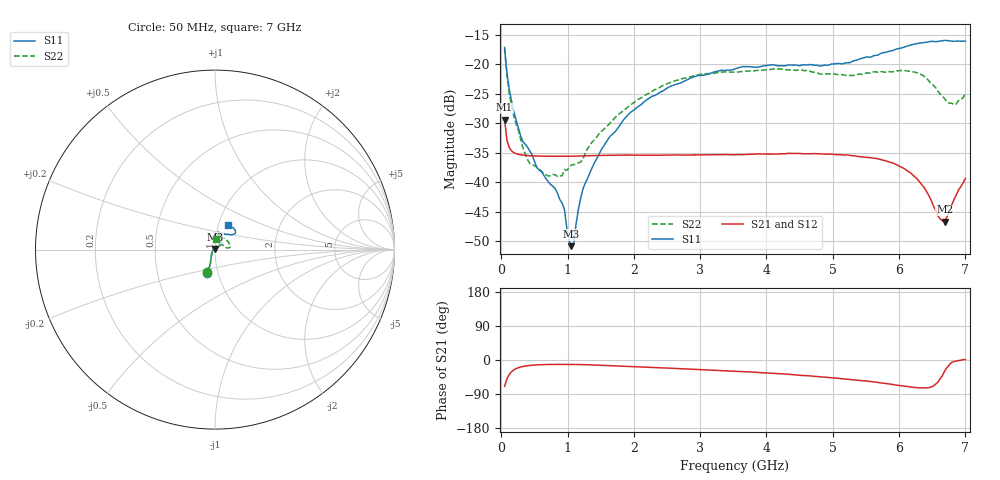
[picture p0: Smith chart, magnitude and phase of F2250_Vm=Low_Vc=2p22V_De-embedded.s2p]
! Integrated Device Technology
! Corporate Headquarters
! 6024 Silver Creek Valley Road
! San Jose, CA 95138  USA
! Phone:  1-408-284-8200
! Toll Free:  1-800-223-1366
! Webpage:  http://www.idt.com/
! Timing and RF Division
! 515 Groton Road, Suite 102
! Westford, MA 01886-6024
! Device:  F2250
! Description: Voltage Variable RF Attenuator
! Frequency:  50.0 -  6000.00 MHz
! Package:  3x3 mm Thin QFN Plastic Package: 16 pin
! Ports:  2 RF, 3 DC
!  Pin  1  = GND
!  Pin  2  = NC
!  Pin  3  = RF1  = Port 1
!  Pin  4  = NC
!  Pin  5  = GND
!  Pin  6  = GND
!  Pin  7  = GND
!  Pin  8  = GND
!  Pin  9  = NC
!  Pin 10  = RF2  = Port 2
!  Pin 11  = NC
!  Pin 12  = GND
!  Pin 13  = GND
!  Pin 14  = VCNTRL
!  Pin 15  = VDD
!  Pin 16  = VMODE
! Vcntrl:  2.220 Volts
! Vmode:  +0.000 Volts
! Vdd:  +3.30  Volts
! Current:  1.177 mA
! Data:  The device was measured on a the F2250 evaluation board which has
!  individual transmission lines to the RF pins.  Data was collected
!  using a calibrated network analyzer.  The evaluation board was
!  de-embedded using a TRL calibration technique.
!  The reference plane is the edge of the package pin.
! Misc:  SN 10
!  Action Tracker AT0258
! Date Measured:  2014-11-26
! Date:  2015-10-15  MJV
! Note:
!  Integrated Device Technology supplies this data as a sample of measured
!  data at the package pin for this product.  Your particular data for this
!  product may vary.
!  Data was taken at 25 degrees C.
!  Integrated Device Technology reserves the right to change this data at anytime.
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# GHz S dB R 50
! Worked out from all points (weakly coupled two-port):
!   201 points, 50 MHz to 7 GHz, reference 50 ohm
!   highest |S21| = -29.39 dB at 50 MHz (marker M1); lowest = -46.7 dB at 6.687 GHz (marker M2)
!   lowest |S11| = -50.8 dB at 1.058 GHz (marker M3), VSWR 1.01, Z = 49.8 + j0.239 ohm
!   |S11| at or under -10 dB: start of sweep to end of sweep
!   |S22| runs from -39.0 to -17.4 dB; largest |S21 - S12| = 5.9e-05
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0.05  -17.18 -108.6  -29.39 -69.5  -29.38 -69.5  -17.38 -110.5
0.08475  -21.44 -107.4  -32.86 -50.1  -32.87 -50.1  -21.91 -109.0
0.15425  -26.23 -116.6  -34.68 -31.0  -34.68 -30.9  -27.12 -120.1
0.29325  -32.19 -127.8  -35.35 -18.4  -35.35 -18.4  -32.74 -133.5
0.3975  -34.09 -141.8  -35.48 -14.9  -35.48 -15.0  -36.19 -157.2
0.71025  -39.94 -168.7  -35.59 -11.8  -35.59 -11.8  -38.94 153.7
0.91875  -43.54 158.0  -35.61 -11.6  -35.60 -11.5  -38.87 127.1
1.023  -49.91 144.0  -35.59 -11.6  -35.59 -11.6  -37.54 108.4
1.05775  -50.81 123.5  -35.59 -11.7  -35.59 -11.7  -37.07 103.0
1.0925  -50.38 89.2  -35.58 -11.8  -35.58 -11.7  -37.00 98.4
1.162  -44.67 56.8  -35.56 -11.9  -35.56 -11.9  -36.69 87.1
1.2315  -41.13 44.4  -35.53 -12.2  -35.53 -12.2  -36.06 77.7
1.6485  -32.11 42.0  -35.44 -14.7  -35.44 -14.7  -29.88 60.5
1.96125  -28.06 42.2  -35.39 -17.3  -35.39 -17.3  -26.81 53.9
2.37825  -24.87 47.3  -35.40 -20.4  -35.40 -20.4  -24.03 54.7
3.525  -20.80 72.5  -35.34 -29.7  -35.33 -29.7  -21.36 73.8
4.7065  -20.17 72.4  -35.14 -42.7  -35.14 -42.8  -21.36 71.7
5.85325  -17.82 40.5  -36.57 -63.4  -36.57 -63.5  -21.26 21.9
6.27025  -16.51 40.1  -39.39 -72.7  -39.41 -72.7  -21.47 8.6
6.68725  -15.99 48.8  -46.69 -29.3  -46.67 -28.8  -25.89 27.6
6.861  -16.13 55.1  -42.16 -2.4  -42.12 -2.5  -26.76 58.0
7  -16.12 63.2  -39.34 1.1  -39.31 0.9  -24.84 83.8
